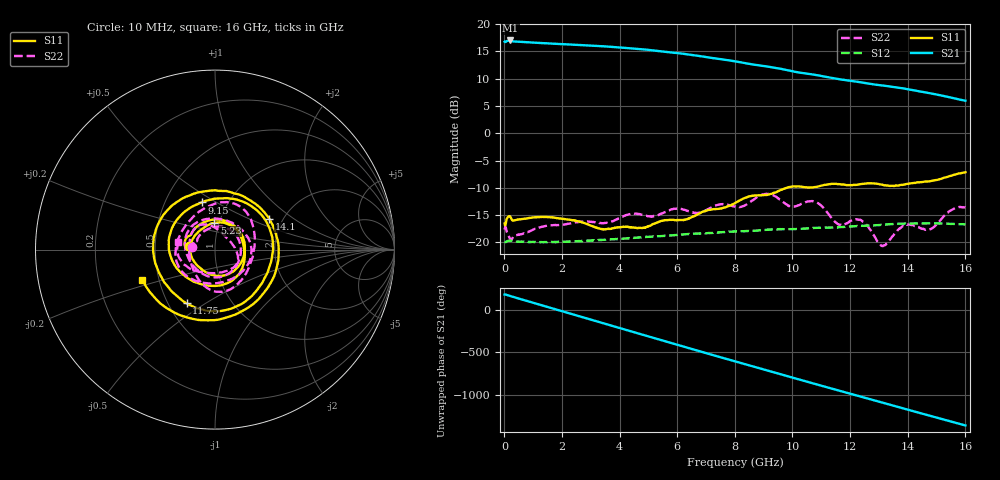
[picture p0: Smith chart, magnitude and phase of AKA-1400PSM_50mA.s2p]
!Keysight Technologies,P9375A,MY57211602,A.15.55.08
!Date: Tuesday, April 18, 2023 17:01:56
!Correction: S11(Cdelta 2-Port  )
!S21(Cdelta 2-Port  )
!S12(Cdelta 2-Port  )
!S22(Cdelta 2-Port  )
!S2P File: Measurements: S11, S21, S12, S22:
# Hz S  dB  R 50
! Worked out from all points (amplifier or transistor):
!   1600 points, 10 MHz to 16 GHz, reference 50 ohm
!   highest |S21| = 17.0 dB at 210 MHz (marker M1)
!   |S21| within 3 dB of that: start of sweep to 6.954 GHz
!   unconditionally stable (mu >= 1): start of sweep to end of sweep
!   at 2.67 GHz: K = 1.07, MAG = 16.3 dB, |S12| = -19.8 dB
!   at 8.01 GHz: K = 1.11, MAG = 13.5 dB, |S12| = -18.0 dB
!   at 16 GHz: K = 1.55, MAG = 7.0 dB, |S12| = -16.7 dB
!   S11 on the Smith chart (normalised r, x): 10 MHz: 0.74, +0.03; 5.23 GHz: 0.95, +0.29; 9.15 GHz: 0.76, +0.43; 11.75 GHz: 0.62, -0.42; 14.1 GHz: 1.71, +0.66; 16 GHz: 0.40, -0.17
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1e7  -16.54 171.3  16.78 175.6  -19.88 -3.7  -17.65 173.8
2.1e8  -15.33 157.0  17.00 158.2  -19.71 -18.2  -19.49 155.5
9.1e8  -15.50 89.7  16.65 88.3  -19.92 -76.2  -17.92 88.9
1.65e9  -15.42 19.5  16.43 15.2  -19.93 -137.0  -16.85 20.2
2.11e9  -15.76 -20.4  16.31 -30.1  -19.88 -174.8  -16.69 -23.6
2.68e9  -16.29 -69.0  16.15 -86.3  -19.77 138.2  -16.23 -72.6
3.26e9  -17.43 -115.0  15.99 -143.5  -19.59 90.1  -16.44 -118.8
3.72e9  -17.49 -148.6  15.83 171.0  -19.42 52.0  -16.20 -160.1
4.48e9  -17.28 147.9  15.52 96.2  -19.20 -11.7  -14.78 137.4
5.23e9  -16.52 91.2  15.14 22.2  -18.90 -74.8  -15.17 65.7
5.34e9  -16.29 81.4  15.07 11.4  -18.88 -84.1  -15.01 53.5
6.42e9  -15.59 -7.4  14.43 -94.6  -18.45 -175.9  -14.30 -47.3
7.21e9  -13.97 -76.8  13.79 -171.9  -18.27 116.1  -13.55 -130.5
8.01e9  -12.77 -146.2  13.18 110.4  -18.01 47.7  -13.48 161.0
9.15e9  -11.28 106.0  12.21 1.3  -17.67 -49.5  -11.11 61.3
9.92e9  -9.83 38.0  11.45 -72.3  -17.57 -116.1  -13.35 -7.4
1.067e10  -9.94 -27.0  10.79 -142.7  -17.39 179.9  -12.45 -78.5
1.175e10  -9.40 -117.9  9.80 115.5  -17.19 86.6  -16.79 174.9
1.334e10  -9.63 101.4  8.61 -33.3  -16.67 -51.4  -19.75 15.8
1.41e10  -9.16 29.4  7.97 -104.9  -16.54 -118.3  -16.75 -38.6
1.494e10  -8.61 -57.0  7.16 176.7  -16.51 168.0  -17.01 -113.7
1.6e10  -7.15 -157.3  5.96 79.0  -16.71 76.1  -13.61 168.2
